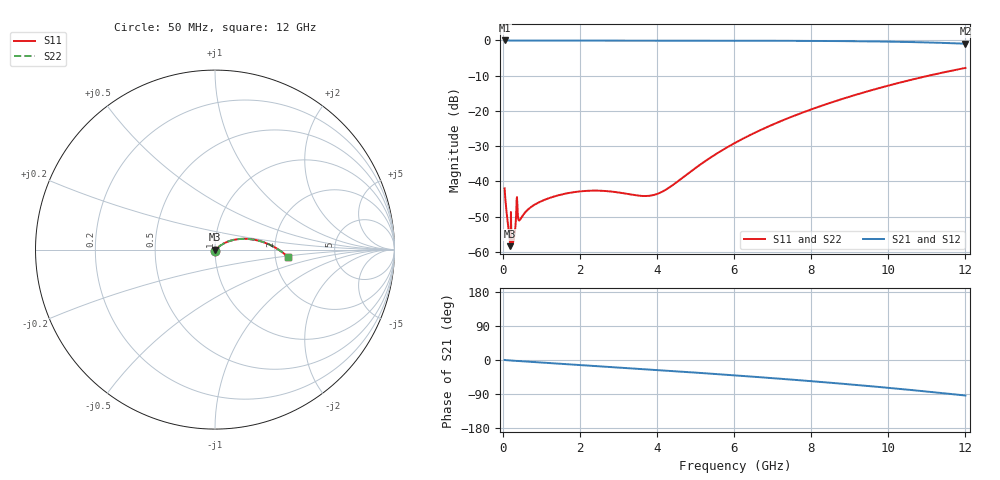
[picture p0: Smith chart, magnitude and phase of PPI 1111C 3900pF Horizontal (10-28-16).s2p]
# MHz S MA R 50
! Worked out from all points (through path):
!   1601 points, 50 MHz to 12 GHz, reference 50 ohm
!   highest |S21| = 0.00 dB at 50 MHz (marker M1); lowest = -0.9 dB at 12 GHz (marker M2)
!   group delay of S21, straight-line fit = 21.2 ps
!   lowest |S11| = -58.4 dB at 199.4 MHz (marker M3), VSWR 1.00, Z = 50.1 - j0.0753 ohm
!   |S11| at or under -10 dB: start of sweep to 11.05 GHz
!   |S22| runs from -58.4 to -7.8 dB; largest |S21 - S12| = 0
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50  0.007946 -87.2  0.9996 0.1  0.9996 0.1  0.007946 -87.2
87.34375  0.004344 -84.4  0.9995 -0.3  0.9995 -0.3  0.004344 -84.4
147.0938  0.002187 -74.6  0.9994 -0.9  0.9994 -0.9  0.002187 -74.6
199.375  0.001203 -38.6  0.999 -1.3  0.999 -1.3  0.001203 -38.6
236.7188  0.001413 -42.6  0.9989 -1.5  0.9989 -1.5  0.001413 -42.6
281.5312  0.001447 -7.5  0.9985 -1.9  0.9985 -1.9  0.001447 -7.5
341.2812  0.002759 20.3  0.9974 -2.3  0.9974 -2.3  0.002759 20.3
401.0312  0.003016 -31.3  0.9973 -2.6  0.9973 -2.6  0.003016 -31.3
460.7812  0.002912 -17.3  0.9971 -3.0  0.9971 -3.0  0.002912 -17.3
737.125  0.00433 -24.3  0.9959 -4.8  0.9959 -4.8  0.00433 -24.3
1162.844  0.005677 -40.1  0.9951 -7.6  0.9951 -7.6  0.005677 -40.1
2044.156  0.00724 -55.3  0.9945 -13.3  0.9945 -13.3  0.00724 -55.3
2686.469  0.007283 -56.1  0.9941 -17.5  0.9941 -17.5  0.007283 -56.1
3649.938  0.006198 -30.5  0.9936 -24.0  0.9936 -24.0  0.006198 -30.5
4038.312  0.006739 -7.1  0.9934 -26.6  0.9934 -26.6  0.006739 -7.1
4359.469  0.008468 10.8  0.9932 -28.8  0.9932 -28.8  0.008468 10.8
5375.219  0.02148 34.8  0.9924 -35.9  0.9924 -35.9  0.02148 34.8
6025  0.03514 37.0  0.9915 -40.6  0.9915 -40.6  0.03514 37.0
6943.656  0.06192 34.9  0.9895 -47.5  0.9895 -47.5  0.06192 34.9
8019.156  0.1059 29.0  0.9849 -56.0  0.9849 -56.0  0.1059 29.0
10013.31  0.2295 13.6  0.9616 -73.6  0.9616 -73.6  0.2295 13.6
12000  0.4074 -5.6  0.8992 -93.7  0.8992 -93.7  0.4074 -5.6
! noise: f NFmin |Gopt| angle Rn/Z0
50  0.0004131  0.8785  0.3385  0.0007356
1372  0.00799  0.8328  9.161  0.01002
2701  0.01195  0.7886  17.91  0.01136
4031  0.01523  0.7626  26.42  0.01235
5360  0.01829  0.7482  34.59  0.01335
6682  0.02127  0.7422  42.31  0.01444
8012  0.02433  0.7427  49.63  0.01571
9341  0.02756  0.7483  56.47  0.01721
1.067e+04  0.03104  0.7579  62.85  0.01903
1.2e+04  0.03489  0.7706  68.78  0.02127
